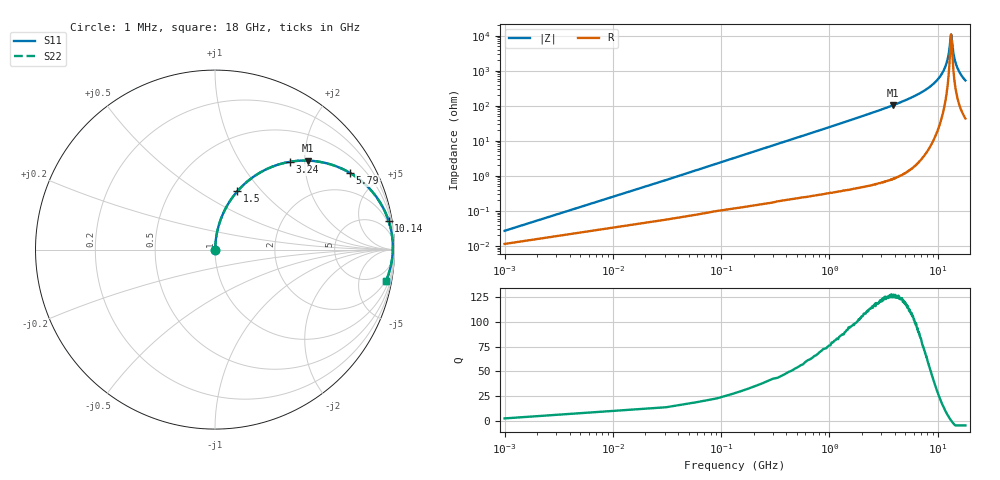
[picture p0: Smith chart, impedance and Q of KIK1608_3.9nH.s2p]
!version-2
!date-01.2022
!Series
# MHz S RI R 50
!Freq ReS11 ImS11 ReS21 ImS21 ReS12 ImS12 ReS22 ImS22
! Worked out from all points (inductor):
!   601 points, 1 MHz to 18 GHz, reference 50 ohm
!   read as one part in series: L = 3.9 nH near 91 MHz
!   highest Q = 127 at 3.87 GHz (marker M1), where L = 4.26 nH
!   self-resonance near 13.26 GHz
!   S11 on the Smith chart (normalised r, x): 1 MHz: 1.00, +0.00; 1.5 GHz: 1.01, +0.75; 3.24 GHz: 1.01, +1.69; 5.79 GHz: 1.03, +3.50; 10.14 GHz: 1, +12; 18 GHz: 2, -11
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1  0.000128 0.000245  0.9999 -0.000245  0.9999 -0.000245  0.000128 0.000245
121  0.002 0.0296  0.998 -0.0296  0.998 -0.0296  0.002 0.0296
181  0.00333 0.0442  0.9967 -0.0442  0.9967 -0.0442  0.00333 0.0442
301  0.00715 0.0731  0.9929 -0.0731  0.9929 -0.0731  0.00715 0.0731
481  0.0159 0.1159  0.9841 -0.1159  0.9841 -0.1159  0.0159 0.1159
751  0.0355 0.1776  0.9645 -0.1776  0.9645 -0.1776  0.0355 0.1776
1500  0.1245 0.3249  0.8755 -0.3249  0.8755 -0.3249  0.1245 0.3249
3030  0.3813 0.4816  0.6187 -0.4816  0.6187 -0.4816  0.3813 0.4816
3240  0.4169 0.489  0.5831 -0.489  0.5831 -0.489  0.4169 0.489
3870  0.5178 0.4957  0.4822 -0.4957  0.4822 -0.4957  0.5178 0.4957
5790  0.7522 0.4271  0.2478 -0.4271  0.2478 -0.4271  0.7522 0.4271
6030  0.7738 0.4135  0.2262 -0.4135  0.2262 -0.4135  0.7738 0.4135
9030  0.9394 0.2271  0.0606 -0.2271  0.0606 -0.2271  0.9394 0.2271
10140  0.9667 0.1614  0.0333 -0.1614  0.0333 -0.1614  0.9667 0.1614
12030  0.9885 0.06  0.0115 -0.06  0.0115 -0.06  0.9885 0.06
12630  0.9906 0.0307  0.0094 -0.0307  0.0094 -0.0307  0.9906 0.0307
13170  0.991 0.00541  0.00904 -0.00541  0.00904 -0.00541  0.991 0.00541
13290  0.9909 -6.1e-05  0.00914 6.1e-05  0.00914 6.1e-05  0.9909 -6.1e-05
14040  0.9889 -0.0331  0.0111 0.0331  0.0111 0.0331  0.9889 -0.0331
15030  0.9833 -0.0736  0.0167 0.0736  0.0167 0.0736  0.9833 -0.0736
16290  0.9722 -0.1207  0.0278 0.1207  0.0278 0.1207  0.9722 -0.1207
18000  0.9517 -0.1771  0.0483 0.1771  0.0483 0.1771  0.9517 -0.1771
